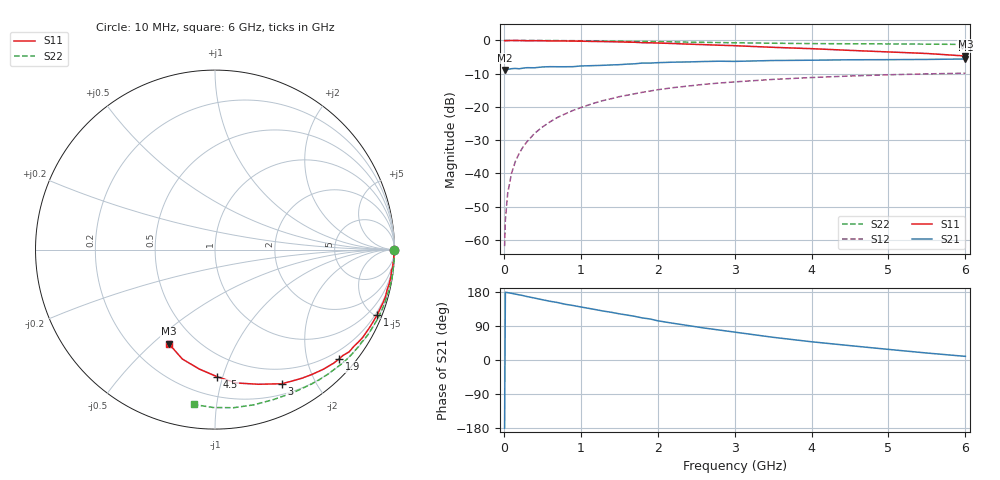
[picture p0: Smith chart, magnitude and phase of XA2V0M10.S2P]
! SIEMENS Discrete & RF Semiconductors
! BFY180
! Si NPN RF Bipolar Junction Transistor in MICRO-X
! VCE = 2 V  IC = 0.1 mA
! Common Emitter S-Parameters:  May  1997
# GHz  S  MA  R  50
!  f  S11  S21  S12  S22
! GHz  MAG  ANG  MAG  ANG  MAG  ANG  MAG  ANG
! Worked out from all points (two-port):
!   36 points, 10 MHz to 6 GHz, reference 50 ohm
!   highest |S21| = -5.58 dB at 6 GHz (marker M1); lowest = -8.9 dB at 10 MHz (marker M2)
!   |S21| within 3 dB of the highest: 82.05 MHz to end of sweep
!   lowest |S11| = -4.7 dB at 6 GHz (marker M3), VSWR 3.80, Z = 17.8 - j28.2 ohm
!   |S11| at or under -10 dB: nowhere
!   |S22| runs from -1.2 to 0.0 dB; largest |S21 - S12| = 0.39
!   S11 on the Smith chart (normalised r, x): 10 MHz: open; 1 GHz: 0.36, -5.17; 1.9 GHz: 0.32, -2.61; 3 GHz: 0.32, -1.57; 4.5 GHz: 0.34, -0.96; 6 GHz: 0.36, -0.56
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0.01  0.9949 -0.1  0.359 -179.9  0.0008 86.4  0.9981 -0.1
0.02  0.9903 -0.5  0.368 178.7  0.002 87.4  0.9999 -0.4
0.05  0.9956 -1.1  0.366 177.8  0.005 83.4  0.999 -1.0
0.1  0.9973 -2.3  0.376 176.0  0.01 87.7  0.9994 -1.9
0.15  0.9999 -3.3  0.379 173.9  0.0151 86.5  0.9999 -2.8
0.2  0.9948 -4.2  0.375 171.9  0.02 86.5  0.9992 -3.8
0.3  0.9899 -6.5  0.389 167.5  0.0298 84.1  0.9985 -5.8
0.4  0.9916 -8.6  0.388 163.4  0.04 82.5  0.9993 -7.6
0.5  0.9893 -11.1  0.399 159.1  0.0496 80.1  0.9979 -9.6
0.7  0.9858 -15.4  0.402 151.6  0.0696 75.9  0.995 -13.4
1  0.9746 -21.8  0.413 140.0  0.0975 69.5  0.9897 -19.2
1.1  0.9694 -24.0  0.416 136.4  0.1068 67.8  0.9872 -21.0
1.5  0.9509 -32.7  0.432 121.9  0.1424 59.4  0.9764 -28.6
1.9  0.9219 -41.4  0.456 108.3  0.1731 51.9  0.9614 -35.8
2.2  0.8992 -47.9  0.471 96.9  0.1947 46.1  0.9534 -41.2
2.6  0.8651 -55.9  0.482 84.5  0.2183 39.0  0.9369 -47.7
3  0.8344 -63.6  0.484 73.6  0.2377 32.2  0.9224 -54.2
3.5  0.788 -72.2  0.499 59.9  0.2593 24.9  0.908 -61.4
4  0.7522 -81.0  0.504 48.1  0.2765 17.6  0.8968 -68.7
4.5  0.709 -88.9  0.512 37.9  0.2915 11.0  0.8917 -75.9
5.5  0.6364 -106.6  0.518 18.4  0.3139 -2.1  0.8799 -90.6
6  0.5835 -116.2  0.526 9.6  0.3214 -8.8  0.8711 -97.9
